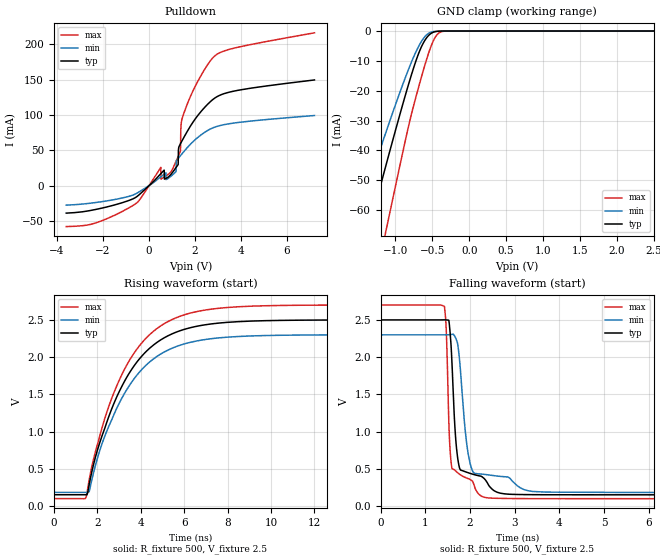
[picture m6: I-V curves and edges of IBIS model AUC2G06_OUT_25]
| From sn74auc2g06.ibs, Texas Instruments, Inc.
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[Model]   AUC2G06_OUT_25
Model_type  Open_drain
Enable   Active-Low
Vref =   0
Rref =   500
Cref =   30p
Vmeas =   1.25
| variable   typ   min   max
C_comp   2.87pF   2.41pF   3.25pF
| C_pulldown   5.35pF   1.05pF   13.60pF
| C_tri-state   2.87pF   2.41pF   3.25pF
[Temperature Range]   40   100   -40
| Ambient temperature   25   85   -40
[Voltage range]   2.5   2.3   2.7
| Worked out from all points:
|   slope of the pulldown table from 0 to 0.375 V, typ, clamps not added: 31 ohm
|   GND clamp passes 1 mA (typ) near -0.53 V on its own axis
|   rising waveform, R_fixture 500, V_fixture 2.5: 20-80 % time 2.22ns typ, 2.22ns min, 2.2ns max; typ from 0.154 V to 2.5 V
|   falling waveform, R_fixture 500, V_fixture 2.5: 20-80 % time 143ps typ, 212ps min, 92.9ps max; typ from 2.5 V to 0.154 V
[GND Clamp]
| AUC2G06_OUT_25
|   Voltage   I(typ)   I(min)   I(max)
-3.6V     -279.3mA   -228.7mA   -348mA
-1.585V   -87.68mA   -68.18mA   -119.7mA
-1.53V    -82.49mA   -63.96mA   -113.4mA
-1.34V    -64.62mA   -49.54mA   -91.44mA
-1.16V    -47.9mA    -36.19mA   -70.6mA
-1.11V    -43.3mA    -32.56mA   -64.8mA
-730mV    -10.56mA   -7.384mA   -22.79mA
-630mV    -4.374mA   -2.805mA   -13.86mA
-530mV    -1.024mA   -505.6uA   -5.921mA
-440mV    -130.5uA   -65.28uA   -1.345mA
-340mV    -7.443uA   -5.464uA   -72.36uA
2.5V      609.9pA    770.4pA    903.3pA
[Pulldown]
| AUC2G06_OUT_25
|   Voltage   I(typ)   I(min)   I(max)
-3.6V     -38.75mA   -27.46mA   -57.79mA
-1.19V    -24.29mA   -17.54mA   -36.85mA
515mV     17.02mA    12.57mA    25.99mA
520mV     17.2mA     12.7mA     9.298mA
930mV     15.04mA    12.66mA    18.59mA
1.27V     30.04mA    38.39mA    41.38mA
1.285V    51.79mA    39.01mA    42.52mA
1.37V     59.36mA    42.45mA    48.97mA
1.41V     61.79mA    44.06mA    89.97mA
1.645V    75.61mA    53.07mA    113.7mA
2.89V     124.5mA    83.14mA    184.2mA
7.2V      149.5mA    99.24mA    216.2mA
[Ramp]
| AUC2G06_OUT_25
| variable   typ   min   max
dV/dt_r   1.41/2.22E-09   1.27/2.22E-09   1.56/2.20E-09
dV/dt_f   1.41/1.45E-10   1.27/2.24E-10   1.56/9.60E-11
R_load = 500
[Rising Waveform]
| AUC2G06_OUT_25
R_fixture =   500
C_fixture =   0
L_fixture =   0
V_fixture =   2.5
V_fixture_min = 2.3
V_fixture_max = 2.7
|   Time   V(typ)   V(min)   V(max)
0s        154.5mV    186.3mV    102.6mV
1.455ns   154.1mV    185.9mV    105mV
1.625ns   285.7mV    195.9mV    349mV
1.905ns   646.8mV    536.5mV    720mV
2.265ns   981mV      875.7mV    1.099V
3.2ns     1.646V     1.485V     1.806V
4.285ns   2.085V     1.902V     2.265V
5.64ns    2.335V     2.142V     2.529V
9.115ns   2.483V     2.284V     2.683V
22ns      2.499V     2.3V       2.7V
[Falling Waveform]
| AUC2G06_OUT_25
R_fixture =   500
C_fixture =   0
L_fixture =   0
V_fixture =   2.5
V_fixture_min = 2.3
V_fixture_max = 2.7
|   Time   V(typ)   V(min)   V(max)
0s        2.5V       2.3V       2.7V
1.425ns   2.501V     2.3V       2.682V
1.47ns    2.5V       2.3V       2.314V
1.525ns   2.495V     2.3V       1.125V
1.59ns    1.983V     2.305V     525.1mV
1.675ns   932.2mV    2.26V      476mV
1.765ns   512.8mV    1.958V     430.6mV
1.995ns   443.1mV    590.9mV    361mV
2.35ns    348.8mV    426.6mV    117.9mV
22ns      154.5mV    186.3mV    102.6mV
